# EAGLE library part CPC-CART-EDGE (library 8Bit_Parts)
CPC+ Cartridge Edge
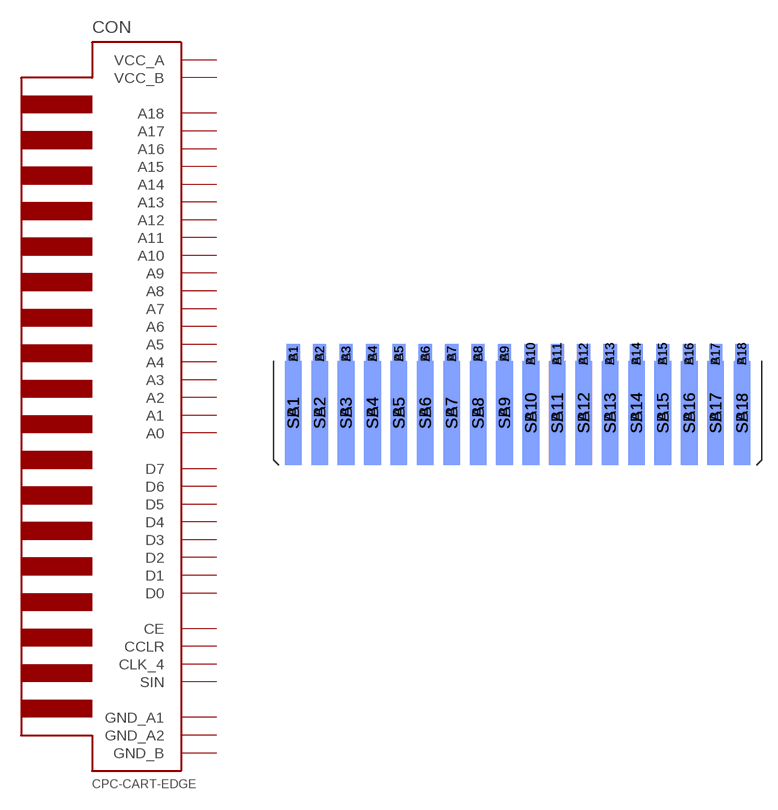
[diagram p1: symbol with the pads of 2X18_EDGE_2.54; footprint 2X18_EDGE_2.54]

Designator prefix CON

## CPC-CART-EDGE  [2X18_EDGE_2.54]
A1  GND_A1
A2  GND_A2
A3  SIN
A4  D2
A5  D1
A6  D0
A7  A0
A8  A1
A9  A2
A10  A3
A11  A11
A12  A9
A13  A8
A14  A13
A15  A14
A16  A17
A17  A18
A18  VCC_A
B1  GND_B
B2  CCLR
B3  D3
B4  D4
B5  D5
B6  D6
B7  D7
B8  CE
B9  A10
B10  A4
B11  A5
B12  A6
B13  A7
B14  A12
B15  A15
B16  A16
B17  CLK_4
B18  VCC_B

## Footprint 2X18_EDGE_2.54 (pad centres in mm)
smd 1.27 x 1.905 bottom: A1 -21.59,5.715; A2 -19.05,5.715; A3 -16.51,5.715; A4 -13.97,5.715; A5 -11.43,5.715; A6 -8.89,5.715; A7 -6.35,5.715; A8 -3.81,5.715; A9 -1.27,5.715; A10 1.27,5.715; A11 3.81,5.715; A12 6.35,5.715; A13 8.89,5.715; A14 11.43,5.715; A15 13.97,5.715; A16 16.51,5.715; A17 19.05,5.715; A18 21.59,5.715
smd 1.27 x 1.905: B1 -21.59,5.715; B2 -19.05,5.715; B3 -16.51,5.715; B4 -13.97,5.715; B5 -11.43,5.715; B6 -8.89,5.715; B7 -6.35,5.715; B8 -3.81,5.715; B9 -1.27,5.715; B10 1.27,5.715; B11 3.81,5.715; B12 6.35,5.715; B13 8.89,5.715; B14 11.43,5.715; B15 13.97,5.715; B16 16.51,5.715; B17 19.05,5.715; B18 21.59,5.715
smd 1.6 x 10 bottom: SA1 -21.59,0; SA2 -19.05,0; SA3 -16.51,0; SA4 -13.97,0; SA5 -11.43,0; SA6 -8.89,0; SA7 -6.35,0; SA8 -3.81,0; SA9 -1.27,0; SA10 1.27,0; SA11 3.81,0; SA12 6.35,0; SA13 8.89,0; SA14 11.43,0; SA15 13.97,0; SA16 16.51,0; SA17 19.05,0; SA18 21.59,0
smd 1.6 x 10: SB1 -21.59,0; SB2 -19.05,0; SB3 -16.51,0; SB4 -13.97,0; SB5 -11.43,0; SB6 -8.89,0; SB7 -6.35,0; SB8 -3.81,0; SB9 -1.27,0; SB10 1.27,0; SB11 3.81,0; SB12 6.35,0; SB13 8.89,0; SB14 11.43,0; SB15 13.97,0; SB16 16.51,0; SB17 19.05,0; SB18 21.59,0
